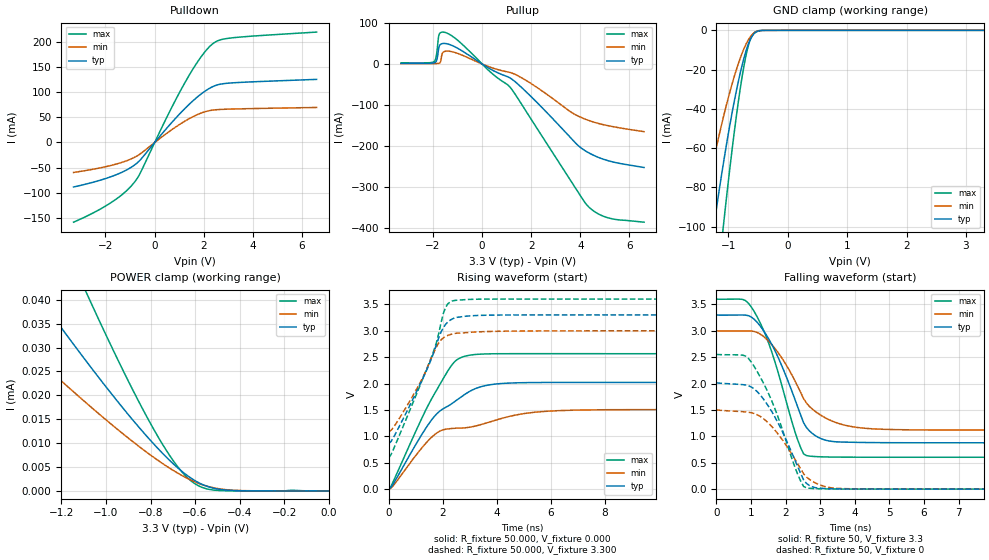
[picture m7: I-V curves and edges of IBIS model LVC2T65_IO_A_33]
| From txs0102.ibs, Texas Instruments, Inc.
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[Model]   LVC2T65_IO_A_33
Model_type  I/O
Vinl=0.15
Vinh=3.2
Enable   Active-High
Vref =   3.3
Rref =   1000000
Cref =   15p
Vmeas =   1.65
| variable   typ   min   max
C_comp   5.16pF   4.52pF   5.65pF
| C_pullup   5.95pF   4.45pF   6.78pF
| C_pulldown   5.65pF   5.18pF   6.69pF
| C_tri-state   5.16pF   4.52pF   5.65pF
[Temperature Range]   40   100   -40
| Ambient temperature   25   85   -40
[Voltage range]   3.3   3   3.6
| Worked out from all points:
|   slope of the pulldown table from 0 to 0.495 V, typ, clamps not added: 17.3 ohm
|   slope of the pullup table from 0 to 0.495 V, typ, clamps not added: 28.5 ohm
|   GND clamp passes 1 mA (typ) near -0.54 V on its own axis
|   rising waveform, R_fixture 50.000, V_fixture 0.000: 20-80 % time 1.81ns typ, 2.75ns min, 1.47ns max; typ from 0.004 V to 2.02 V
|   falling waveform, R_fixture 50, V_fixture 3.3: 20-80 % time 924ps typ, 1.1ns min, 849ps max; typ from 3.3 V to 0.877 V
|   rising waveform, R_fixture 50.000, V_fixture 3.300: 20-80 % time 1.26ns typ, 1.14ns min, 1.33ns max; typ from 0.867 V to 3.3 V
|   falling waveform, R_fixture 50, V_fixture 0: 20-80 % time 902ps typ, 932ps min, 885ps max; typ from 2.01 V to 0.004 V
[GND Clamp]
| LVC2T65_IO_A_33
|   Voltage   I(typ)   I(min)   I(max)
-3.3V     -657.4mA   -474.3mA   -883.2mA
-1.46V    -148.2mA   -98.4mA    -216mA
-1.245V   -100.3mA   -65.89mA   -147.6mA
-1.085V   -68.29mA   -44.57mA   -100.4mA
-890mV    -34.76mA   -22.61mA   -49.73mA
-815mV    -23.92mA   -15.6mA    -33.09mA
-745mV    -15.16mA   -9.985mA   -19.69mA
-690mV    -9.439mA   -6.356mA   -11.22mA
-630mV    -4.725mA   -3.34mA    -4.746mA
-580mV    -2.197mA   -1.659mA   -1.773mA
-525mV    -754.6uA   -628.9uA   -451.7uA
3.3V      340.3pA    12.59nA    82.16pA
[POWER Clamp]
| LVC2T65_IO_A_33
|   Voltage   I(typ)   I(min)   I(max)
-3.3V     184.6uA    122.5uA    302.4uA
-1.64V    63.18uA    42.19uA    101.5uA
-1.59V    59.78uA    39.94uA    95.82uA
-1.315V   41.49uA    27.87uA    65.4uA
-1.11V    28.46uA    19.28uA    43.74uA
-1.06V    25.39uA    17.26uA    38.63uA
-900mV    15.99uA    11.07uA    23.02uA
-760mV    8.55uA     6.184uA    10.84uA
-675mV    4.721uA    3.651uA    4.882uA
-615mV    2.576uA    2.191uA    1.979uA
-460mV    171.3nA    257.9nA    30.51nA
0V        0A         0A         0A
[Pulldown]
| LVC2T65_IO_A_33
|   Voltage   I(typ)   I(min)   I(max)
-3.3V     -88.33mA   -59.48mA   -158.2mA
-1.815V   -68.6mA    -46.05mA   -120.7mA
-1.255V   -57.38mA   -38.25mA   -100.7mA
-840mV    -45.53mA   -30.03mA   -80.1mA
-580mV    -34.48mA   -22.51mA   -60.36mA
515mV     29.43mA    18.89mA    51.68mA
1.235V    67.44mA    42.37mA    118.7mA
1.895V    96.3mA     58.39mA    170.1mA
2.395V    111.4mA    64.48mA    196.9mA
2.725V    116.2mA    65.7mA     204.4mA
3.235V    118.6mA    66.53mA    208.2mA
6.6V      125.3mA    69.57mA    219.2mA
[Pullup]
| LVC2T65_IO_A_33
|   Voltage   I(typ)   I(min)   I(max)
-3.3V     1.645mA    885.5uA    2.693mA
-1.96V    2.762mA    912.2uA    5.543mA
-1.865V   6.675mA    1.017mA    19.49mA
-1.775V   35.42mA    1.376mA    65.28mA
-1.73V    45.28mA    2.056mA    74.27mA
-1.59V    50.05mA    28.42mA    77.9mA
-1.225V   45.24mA    30.04mA    68.52mA
1.15V     -34.49mA   -20.89mA   -57.45mA
3.905V    -198.7mA   -126.9mA   -312.3mA
4.355V    -217.3mA   -138.1mA   -349.7mA
5.12V     -236mA     -150.5mA   -375.5mA
6.6V      -252.8mA   -165.3mA   -386.4mA
[Ramp]
| LVC2T65_IO_A_33
| variable   typ   min   max
dV/dt_r   1.27/1.82E-09   0.95/2.78E-09   1.58/1.48E-09
dV/dt_f   1.45/9.24E-10   1.14/1.10E-09   1.80/8.49E-10
R_load = 50
[Rising Waveform]
R_fixture = 50.000
V_fixture = 0.000
V_fixture_min = 0.000
V_fixture_max = 0.000
C_fixture = 0.000
L_fixture = 0.000
|  time   V(typ)   V(min)   V(max)
0s        4.04mV     3.467mV    4.476mV
1.596ns   1.323V     991.8mV    1.724V
1.932ns   1.498V     1.112V     2.023V
2.352ns   1.628V     1.152V     2.365V
2.856ns   1.81V      1.166V     2.524V
3.864ns   1.987V     1.294V     2.565V
4.872ns   2.017V     1.422V     2.567V
5.88ns    2.022V     1.478V     2.567V
9.912ns   2.023V     1.509V     2.566V
419.9ns   2.015V     1.503V     2.555V
[Falling Waveform]
| LVC2T65_IO_A_33
R_fixture =   50
C_fixture =   0
L_fixture =   0
V_fixture =   3.3
V_fixture_min = 3
V_fixture_max = 3.6
|   Time   V(typ)   V(min)   V(max)
0s        3.3V       3V         3.6V
756ps     3.298V     2.997V     3.594V
1.092ns   3.218V     2.987V     3.365V
1.764ns   2.525V     2.604V     2.257V
2.268ns   1.706V     2.057V     1.095V
2.52ns    1.262V     1.717V     670.8mV
2.856ns   1.017V     1.476V     620.4mV
3.444ns   900.1mV    1.266V     610.1mV
10.92ns   880.6mV    1.118V     607mV
419.9ns   876.9mV    1.105V     606.1mV
[Rising Waveform]
R_fixture = 50.000
V_fixture = 3.300
V_fixture_min = 3.000
V_fixture_max = 3.600
C_fixture = 0.000
L_fixture = 0.000
|  time   V(typ)   V(min)   V(max)
0s        867.2mV    1.093V     599.9mV
252ps     1.06V      1.234V     857.8mV
840ps     1.655V     1.728V     1.575V
1.596ns   2.497V     2.509V     2.53V
1.848ns   2.869V     2.771V     2.951V
2.016ns   3.057V     2.865V     3.324V
2.1ns     3.12V      2.893V     3.44V
2.352ns   3.225V     2.939V     3.564V
3.36ns    3.291V     2.981V     3.598V
419.9ns   3.3V       3V         3.6V
[Falling Waveform]
| LVC2T65_IO_A_33
R_fixture =   50
C_fixture =   0
L_fixture =   0
V_fixture =   0
V_fixture_min = 0
V_fixture_max = 0
|   Time   V(typ)   V(min)   V(max)
0s        2.014V     1.501V     2.554V
756ps     1.981V     1.469V     2.54V
924ps     1.961V     1.459V     2.477V
1.26ns    1.791V     1.383V     2.134V
1.596ns   1.477V     1.192V     1.68V
2.268ns   556.4mV    573.2mV    421.9mV
2.52ns    179.9mV    295.6mV    54.98mV
2.772ns   47.29mV    153.5mV    16.61mV
3.276ns   12.98mV    33.38mV    7.434mV
419.9ns   3.94mV     3.324mV    4.391mV
